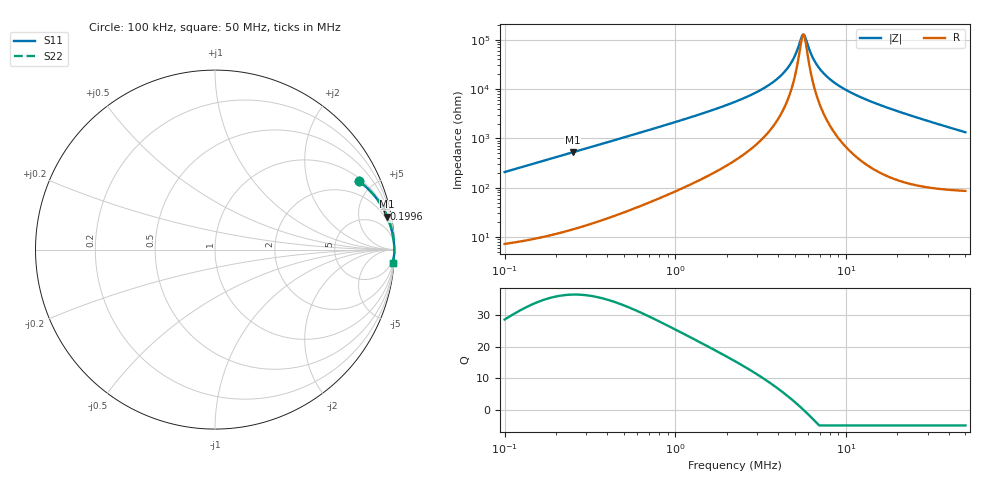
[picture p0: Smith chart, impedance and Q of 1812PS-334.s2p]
# MHz S MA R 50
!Freq  MagS11  AngS11  MagS21  AngS21  MagS12  AngS12  MagS22  AngS22
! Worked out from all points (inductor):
!   801 points, 100 kHz to 50 MHz, reference 50 ohm
!   read as one part in series: L = 330 uH near 103.2 kHz
!   highest Q = 36.5 at 250.1 kHz (marker M1), where L = 331 uH
!   self-resonance near 5.592 MHz
!   S11 on the Smith chart (normalised r, x): 100 kHz: 1.14, +4.15; 199.6 kHz: 1.23, +8.29; 50 MHz: 3, -27
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0.1  0.8888 25.3  0.4283 -62.7  0.4283 -62.7  0.8888 25.3
0.1996459  0.966 13.5  0.233 -74.9  0.233 -74.9  0.966 13.5
0.250091  0.977 10.8  0.188 -77.6  0.188 -77.6  0.977 10.8
0.2831897  0.9814 9.6  0.1667 -78.8  0.1667 -78.8  0.9814 9.6
0.7957584  0.9961 3.4  0.05919 -84.6  0.05919 -84.6  0.9961 3.4
2.236068  0.9987 1.0  0.01817 -85.2  0.01817 -85.2  0.9987 1.0
3.246558  0.999 0.6  0.009936 -83.8  0.009936 -83.8  0.999 0.6
3.733791  0.9991 0.4  0.007267 -82.3  0.007267 -82.3  0.9991 0.4
4.162766  0.9991 0.3  0.005298 -80.2  0.005298 -80.2  0.9991 0.3
4.499032  0.9991 0.2  0.00394 -77.3  0.00394 -77.3  0.9991 0.2
4.824836  0.9992 0.2  0.002754 -72.4  0.002754 -72.4  0.9992 0.2
5.094464  0.9992 0.1  0.001872 -64.3  0.001872 -64.3  0.9992 0.1
5.463387  0.9992 0.0  0.0009279 -31.6  0.0009279 -31.6  0.9992 0.0
5.592205  0.9992 0.0  0.0007891 -6.3  0.0007891 -6.3  0.9992 0.0
5.7687  0.9992 -0.0  0.0008959 29.9  0.0008959 29.9  0.9992 -0.0
6.332315  0.9992 -0.1  0.002185 69.6  0.002185 69.6  0.9992 -0.1
6.738328  0.9993 -0.2  0.003215 76.4  0.003215 76.4  0.9993 -0.2
7.226293  0.9993 -0.2  0.004416 80.2  0.004416 80.2  0.9993 -0.2
8.843662  0.9992 -0.5  0.008073 84.4  0.008073 84.4  0.9992 -0.5
11.78853  0.9991 -0.8  0.01391 86.1  0.01391 86.1  0.9991 -0.8
17.7937  0.9987 -1.4  0.02443 86.3  0.02443 86.3  0.9987 -1.4
50  0.9924 -4.3  0.07468 82.0  0.07468 82.0  0.9924 -4.3
